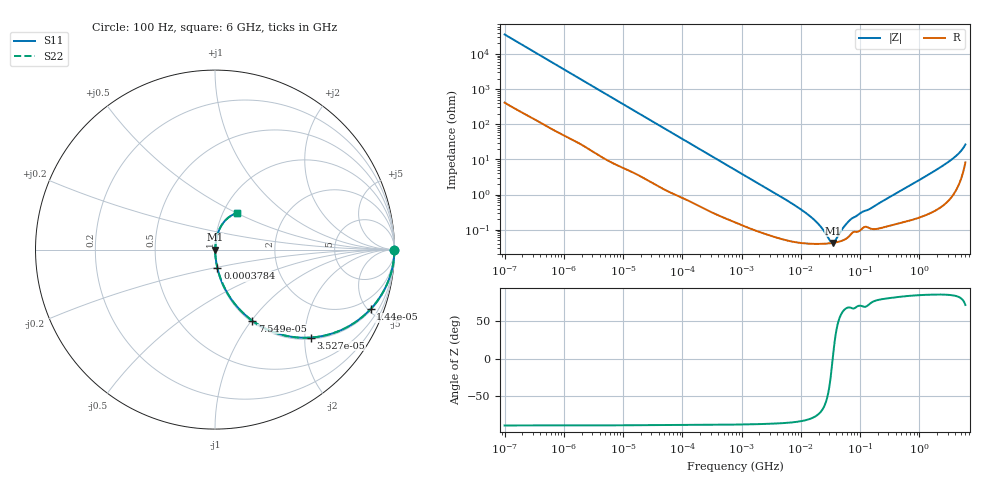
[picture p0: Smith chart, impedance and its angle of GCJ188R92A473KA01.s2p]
!Murata Part Number: GCJ188R92A473KA01
!These Parameters are Measured in Series Mode Connection
!Data Generated on Mar 13, 2026
!  o--ll--o
!Port1  Port2
!  o------o
!Operation Temp=25[degC], DC Bias Voltage=0[V]
!Freq. Start=100[Hz] Stop=6[GHz] 401[Steps]
# Hz S RI R 50
!Freq.(Hz) S11(Real) S11(Imag) S21(Real) S21(Imag) S12(Real) S12(Imag) S22(Real) S22(Imag)
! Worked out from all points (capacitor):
!   401 points, 100 Hz to 6 GHz, reference 50 ohm
!   read as one part in series: C = 44.2 nF near 109 Hz
!   lowest |Z| = 42 mohm at 34.83 MHz (marker M1)
!   series resonance near 34.56 MHz, so ESL is about 480 pH
!   S11 on the Smith chart (normalised r, x): 100 Hz: open; 14.4 kHz: 1.09, -5.20; 35.27 kHz: 1.04, -2.14; 75.5 kHz: 1.02, -1.01; 378.4 kHz: 1.01, -0.21; 6 GHz: 1.16, +0.51
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100  1 -0.00278  3.98e-05 0.00278  3.98e-05 0.00278  1 -0.00278
2008  0.9963 -0.0543  0.00374 0.0543  0.00374 0.0543  0.9963 -0.0543
5625  0.9756 -0.1475  0.0244 0.1475  0.0244 0.1475  0.9756 -0.1475
14402  0.867 -0.3314  0.133 0.3314  0.133 0.3314  0.867 -0.3314
35265  0.5343 -0.4901  0.4657 0.4901  0.4657 0.4901  0.5343 -0.4901
40335  0.4691 -0.4902  0.5309 0.4902  0.5309 0.4902  0.4691 -0.4902
75495  0.2077 -0.396  0.7923 0.396  0.7923 0.396  0.2077 -0.396
147774  0.0682 -0.241  0.9318 0.241  0.9318 0.241  0.0682 -0.241
378399  0.0131 -0.1013  0.9869 0.1013  0.9869 0.1013  0.0131 -0.1013
774597  0.00418 -0.0505  0.9958 0.0505  0.9958 0.0505  0.00418 -0.0505
6353432  0.000515 -0.00621  0.9995 0.00621  0.9995 0.00621  0.000515 -0.00621
1.555665e7  0.000399 -0.00211  0.9996 0.00211  0.9996 0.00211  0.000399 -0.00211
2.225763e7  0.000395 -0.00108  0.9996 0.00108  0.9996 0.00108  0.000395 -0.00108
3.184506e7  0.000412 -0.000196  0.9996 0.000196  0.9996 0.000196  0.000412 -0.000196
3.482834e7  0.00042 1.88e-05  0.9996 -1.88e-05  0.9996 -1.88e-05  0.00042 1.88e-05
3.80911e7  0.000431 0.000234  0.9996 -0.000234  0.9996 -0.000234  0.000431 0.000234
5.449875e7  0.00052 0.00114  0.9995 -0.00114  0.9995 -0.00114  0.00052 0.00114
7.129496e7  0.000766 0.00189  0.9992 -0.00189  0.9992 -0.00189  0.000766 0.00189
3.124326e8  0.00136 0.00827  0.9986 -0.00827  0.9986 -0.00827  0.00136 0.00827
2.679998e9  0.0102 0.0703  0.9898 -0.0703  0.9898 -0.0703  0.0102 0.0703
4.586474e9  0.0372 0.1364  0.9628 -0.1364  0.9628 -0.1364  0.0372 0.1364
6e9  0.1235 0.2046  0.8765 -0.2046  0.8765 -0.2046  0.1235 0.2046
